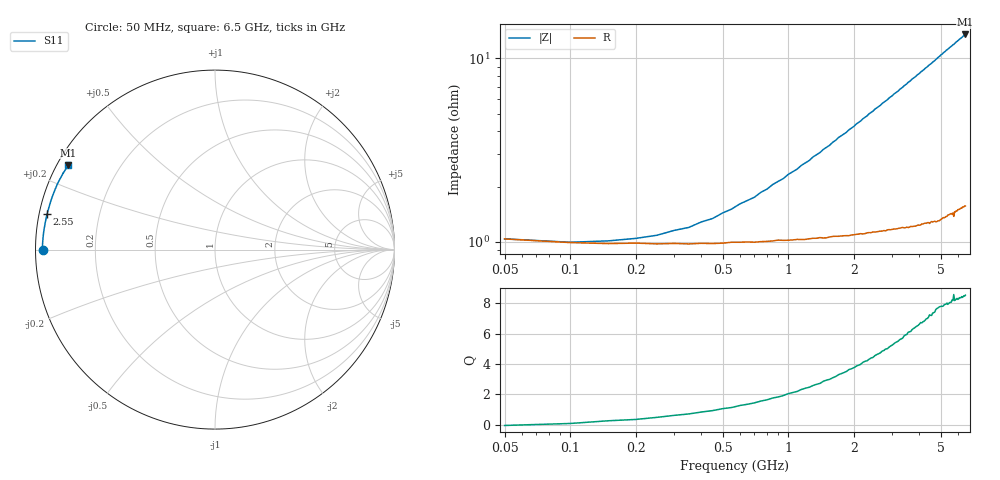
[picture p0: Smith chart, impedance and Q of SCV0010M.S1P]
! Infineon Technologies  Discrete & RF Semiconductors
! BAR63-02L
! Si PIN Diode in TSLP-2
! IF = 10 mA
! S-Parameters:  March  2002
# GHz  S  MA  R  50
!  f  S11
! GHz  MAG  ANG
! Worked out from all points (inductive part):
!   130 points, 50 MHz to 6.5 GHz, reference 50 ohm
!   read as one part to ground: L = 327 pH near 1.6 GHz
!   highest Q = 8.54 at 6.5 GHz (marker M1), where L = 328 pH
!   S11 on the Smith chart (normalised r, x): 50 MHz: 0.02, -0.00; 2.55 GHz: 0.02, +0.11; 6.5 GHz: 0.03, +0.27
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0.05  0.9593 -179.9
0.15  0.9616 179.4
0.2  0.9614 179.2
0.3  0.9615 178.6
0.9  0.96 175.7
1.4  0.9588 173.4
1.45  0.959 173.1
1.55  0.9585 172.7
1.7  0.9582 171.9
1.85  0.9579 171.3
1.9  0.9579 171.0
2.45  0.9561 168.5
2.5  0.9561 168.2
2.55  0.9561 168.0
3.3  0.9541 164.6
3.7  0.9537 162.7
3.85  0.9535 162.1
4.1  0.9524 160.9
4.4  0.9518 159.5
4.55  0.9513 158.9
4.9  0.9511 157.2
5.3  0.9488 155.3
5.65  0.9477 153.8
5.7  0.947 153.5
5.75  0.9492 153.4
5.8  0.9462 153.1
6.1  0.945 151.7
6.5  0.9431 150.0
